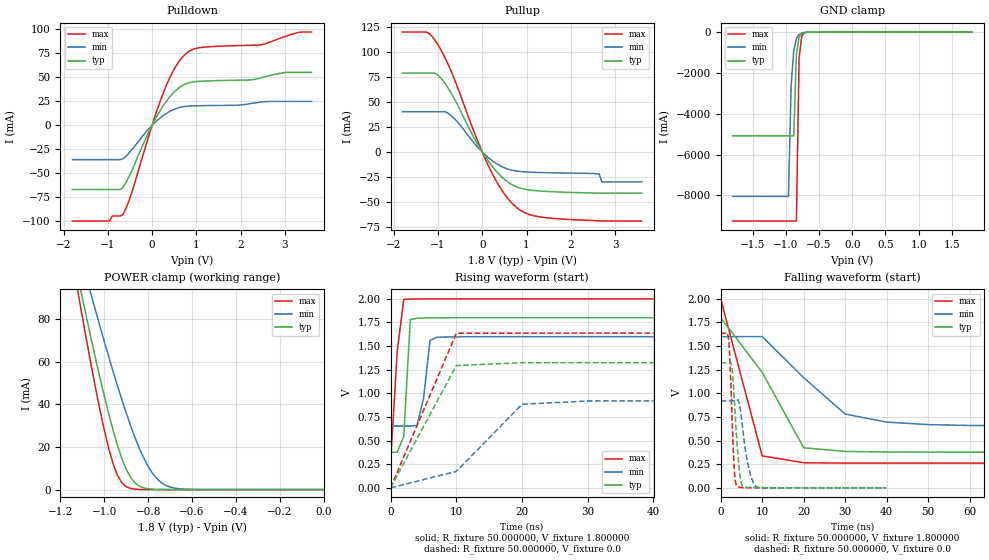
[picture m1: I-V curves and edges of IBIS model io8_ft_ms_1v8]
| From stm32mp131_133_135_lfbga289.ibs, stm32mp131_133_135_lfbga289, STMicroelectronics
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|   Model io8_ft_ms_1v8
[Model]  io8_ft_ms_1v8
Model_type I/O
Polarity   Non-Inverting
Enable   Active-Low
Vinl =   0.540000V
Vinh =   1.260000V
Vmeas =  0.900000V
Cref =   50.000000pF
Rref =   100.000000M
Vref =   0.0V
C_comp   3.181500pF   3.164300pF   3.208900pF
[Temperature Range]   25.000000   0.140000k   -40.000000
[Pullup Reference]   1.800000V   1.600000V   2.000000V
[Pulldown Reference]   0.0V   0.0V   0.0V
[POWER Clamp Reference]   1.800000V   1.600000V   2.000000V
[GND Clamp Reference]   0.0V   0.0V   0.0V
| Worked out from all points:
|   slope of the pulldown table from 0 to 0.27 V, typ, clamps not added: 12.5 ohm
|   slope of the pullup table from 0 to 0.27 V, typ, clamps not added: 16 ohm
|   GND clamp passes 1 mA (typ) near -0.47 V on its own axis
|   POWER clamp passes 1 mA (typ) near -0.83 V on its own axis
|   rising waveform, R_fixture 50.000000, V_fixture 1.800000: 20-80 % time 691ps typ, 1.1ns min, 1.1ns max; typ from 0.377 V to 1.8 V
|   rising waveform, R_fixture 50.000000, V_fixture 0.0: 20-80 % time 6.15ns typ, 7.77ns min, 6.01ns max; typ from 0 V to 1.32 V
|   falling waveform, R_fixture 50.000000, V_fixture 1.800000: 20-80 % time 12.1ns typ, 14ns min, 6.28ns max; typ from 1.8 V to 0.377 V
|   falling waveform, R_fixture 50.000000, V_fixture 0.0: 20-80 % time 1.22ns typ, 1.91ns min, 860ps max; typ from 1.32 V to 0 V
[Pulldown]
|Voltage   I(typ)   I(min)   I(max)
-1.8V     -67.09mA   -35.91mA   -100mA
-960mV    -67.09mA   -35.91mA   -100mA
-900mV    -67.09mA   -35.91mA   -94.73mA
-660mV    -64.86mA   -35.04mA   -93.29mA
-480mV    -49.73mA   -26.7mA    -73.15mA
-60mV     -5.61mA    -2.937mA   -8.854mA
240mV     19.58mA    9.767mA    32.18mA
540mV     36.57mA    17.36mA    61.85mA
780mV     43.58mA    19.81mA    75.41mA
1.14V     46.02mA    20.44mA    81.32mA
2.46V     49.57mA    24.16mA    83.94mA
3.6V      55.18mA    24.86mA    97.31mA
[Pullup]
|Voltage   I(typ)   I(min)   I(max)
-1.8V     79.18mA    40.38mA    120.4mA
-1.26V    79.18mA    40.38mA    120.4mA
-1.02V    77.84mA    40.38mA    109.1mA
-660mV    55.94mA    34.87mA    76.58mA
-180mV    13.76mA    8.769mA    19.71mA
180mV     -11.78mA   -7.161mA   -17.58mA
480mV     -26.67mA   -15.47mA   -40.89mA
780mV     -35.14mA   -19.2mA    -55.89mA
1.44V     -39.57mA   -20.76mA   -65.96mA
2.64V     -41.3mA    -22mA      -69.09mA
2.7V      -41.3mA    -30mA      -69.18mA
3.6V      -41.3mA    -30mA      -69.3mA
[GND_clamp]
|Voltage   I(typ)   I(min)   I(max)
-1.8V     -5.08A     -8.044A    -9.251A
-960mV    -5.08A     -8.044A    -9.251A
-920mV    -5.08A     -2.669A    -9.251A
-880mV    -5.08A     -908mA     -9.251A
-840mV    -1.096A    -323.6mA   -9.251A
-800mV    -248.9mA   -123.7mA   -1.293A
-760mV    -64.81mA   -51.32mA   -196.6mA
-720mV    -22.13mA   -23.23mA   -39.69mA
-480mV    -1.149mA   -1.898mA   -936.1uA
1.8V      0A         44.33nA    0A
[POWER_clamp]
|Voltage   I(typ)   I(min)   I(max)
-1.8V     460.5mA    392.1mA    526.9mA
-1.12V    99.56mA    114.1mA    92.51mA
-1.1V     89.79mA    106.4mA    80.86mA
-1.06V    70.71mA    91.32mA    58.34mA
-1V       43.82mA    69.37mA    27.91mA
-960mV    27.85mA    55.39mA    12.18mA
-900mV    9.544mA    35.9mA     1.368mA
-860mV    3.133mA    24.42mA    203.6uA
-800mV    367uA      10.84mA    10.43uA
-760mV    78.93uA    5.095mA    1.426uA
-700mV    7.679uA    1.212mA    72.45nA
0V        0A         59.16nA    0A
[Ramp]
| variable   typ   min   max
dV/dt_r  0.79476/2.06580n   0.55241/5.06440n   0.98226/1.12831n
dV/dt_f  0.85363/4.36317n   0.56724/10.83154n   1.04297/2.49422n
R_load = 50.000000
[Rising Waveform]
R_fixture= 50.000000
V_fixture= 1.800000
V_fixture_min= 1.600000
V_fixture_max= 2.000000
|time   V(typ)   V(min)   V(max)
0s        377.3mV    654.6mV    261.4mV
1.001ns   376.7mV    654.6mV    1.433V
2.002ns   542.5mV    654.6mV    1.994V
3.003ns   1.78V      654.4mV    1.998V
4.004ns   1.795V     659.1mV    1.999V
5.005ns   1.797V     940mV      2V
6.006ns   1.798V     1.56V      2V
7.007ns   1.799V     1.593V     2V
16.02ns   1.8V       1.6V       2V
99.1ns    1.8V       1.6V       2V
[Rising Waveform]
R_fixture= 50.000000
V_fixture= 0.0
V_fixture_min= 0.0
V_fixture_max= 0.0
|time   V(typ)   V(min)   V(max)
0s        2.004nV    378.7nV    939.1pV
10.01ns   1.294V     173.6mV    1.637V
20.02ns   1.325V     884.8mV    1.637V
30.03ns   1.325V     919.2mV    1.637V
991ns     1.325V     920.7mV    1.637V
[Falling Waveform]
R_fixture= 50.000000
V_fixture= 1.800000
V_fixture_min= 1.600000
V_fixture_max= 2.000000
|time   V(typ)   V(min)   V(max)
0s        1.8V       1.6V       2V
10.01ns   1.222V     1.601V     338.2mV
20.02ns   423.8mV    1.165V     266.1mV
30.03ns   385.6mV    781.1mV    262mV
40.04ns   379.1mV    695.2mV    261.5mV
50.05ns   377.6mV    669.3mV    261.4mV
60.06ns   377.3mV    660.4mV    261.4mV
100.1ns   377.3mV    654.7mV    261.4mV
991ns     377.3mV    654.6mV    261.4mV
[Falling Waveform]
R_fixture= 50.000000
V_fixture= 0.0
V_fixture_min= 0.0
V_fixture_max= 0.0
|time   V(typ)   V(min)   V(max)
0s        1.325V     920.7mV    1.637V
1.922ns   1.324V     920.7mV    1.556V
2.162ns   1.327V     920.7mV    1.412V
2.643ns   1.286V     920.7mV    869.4mV
3.203ns   988.1mV    920.5mV    253.4mV
4.004ns   433.2mV    929.9mV    15.86mV
5.125ns   29.56mV    696.3mV    3.175mV
6.727ns   3.668mV    221.8mV    1.129mV
8.569ns   1.721mV    11.47mV    621.7uV
39.88ns   2.004nV    378.7nV    939.1pV
